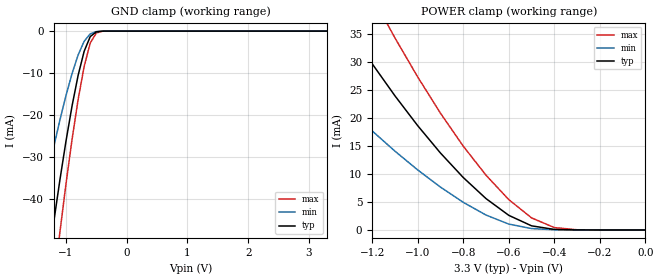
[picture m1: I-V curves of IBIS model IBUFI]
| IBIS file ibufi.ibs created by s2ibis2 version 1.1
| North Carolina State University Electronics Research Laboratory  1995
[IBIS ver]   2.1
[File name]   ibufi.ibs
[File Rev]   1.0
[Date]   Thursday, March 30, 2000
[Source]   From silicon level SPICE at TOSHIBA.
[Notes]   This model does not include the values of Package Model
[Disclaimer]   None.
[Copyright]   Copyright(C) TOSHIBA Corp. 1996-2000. All Rights Reserved
|   Component TC260C
[Component]   TC260C
[Manufacturer]   TOSHIBA
[Package]
| variable   typ   min   max
R_pkg   1.0000f   NA   NA
L_pkg   1.0000fH   NA   NA
C_pkg   1.0000fF   NA   NA
[Pin]  signal_name   model_name   R_pin   L_pin   C_pin
A   A   IBUFI
VDDS   VDDS   POWER
VSS   VSS   GND
| Models and submodels in the file (1): IBUFI (Input)
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|   Model IBUFI
[Model]   IBUFI
Model_type   Input
Polarity   Non-Inverting
Vinl =   0.6600V
Vinh =   2.6400V
C_comp   4.3000pF   NA   NA
|Variable   typ   min   max
[Voltage range]  3.3   3.0   3.6
[Temperature Range]   25.0000   100.0000   0.000
[POWER Clamp Reference]   3.3000V   3.0000V   3.6000V
[GND Clamp Reference]   0.000V   0.000V   0.000V
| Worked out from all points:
|   GND clamp passes 1 mA (typ) near -0.57 V on its own axis
|   POWER clamp passes 1 mA (typ) near -0.51 V on its own axis
[GND_clamp]
| voltage   I(typ)   I(min)   I(max)
-3.3V     -292.8mA   -217.8mA   -337.5mA
-1.5V     -77.97mA   -49.07mA   -98.95mA
-1.3V     -55.88mA   -34.36mA   -72.74mA
-1.2V     -45.43mA   -27.57mA   -60.12mA
-1.1V     -35.51mA   -21.22mA   -47.98mA
-900mV    -17.87mA   -10.14mA   -25.85mA
-800mV    -10.56mA   -5.698mA   -16.34mA
-700mV    -4.792mA   -2.412mA   -8.394mA
-600mV    -1.302mA   -649uA     -2.833mA
-500mV    -170.7uA   -108.2uA   -443.3uA
-400mV    -13.58uA   -13.64uA   -33.16uA
3.3V      153.9pA    4.45uA     -1.048nA
[POWER_clamp]
| voltage   I(typ)   I(min)   I(max)
-3.3V     189.1mA    135.9mA    229.2mA
-1.7V     62.57mA    39.06mA    82.98mA
-1.6V     55.54mA    34.4mA     74.31mA
-1.3V     35.75mA    21.56mA    49.45mA
-1.2V     29.69mA    17.7mA     41.7mA
-1.1V     23.96mA    14.08mA    34.3mA
-900mV    13.74mA    7.658mA    20.85mA
-800mV    9.367mA    4.936mA    14.97mA
-600mV    2.612mA    1.048mA    5.42mA
-500mV    737.5uA    251.8uA    2.156mA
-400mV    94.87uA    37.87uA    425.3uA
0V        153.9pA    711.8pA    166.4pA
